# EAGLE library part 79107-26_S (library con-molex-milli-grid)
RECEPTACAL
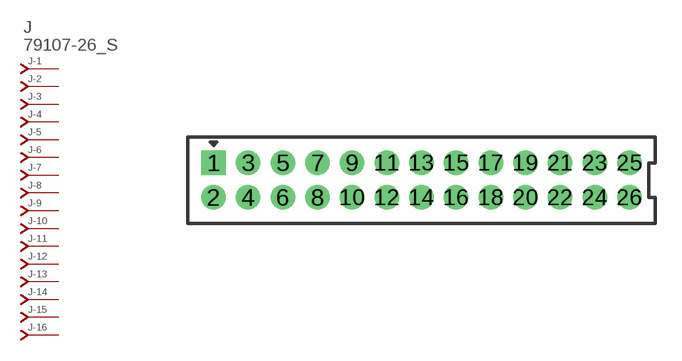
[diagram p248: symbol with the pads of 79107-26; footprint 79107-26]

Designator prefix J; gates -1=J-NV -2=J-N -3=J-N -4=J-N -5=J-N -6=J-N -7=J-N -8=J-N -9=J-N -10=J-N -11=J-N -12=J-N -13=J-N -14=J-N -15=J-N -16=J-N -17=J-N -18=J-N -19=J-N -20=J-N -21=J-N -22=J-N -23=J-N -24=J-N -25=J-N -26=J-N

## 79107-26_S  [79107-26]
1  -1:J  pas
2  -2:J  pas
3  -3:J  pas
4  -4:J  pas
5  -5:J  pas
6  -6:J  pas
7  -7:J  pas
8  -8:J  pas
9  -9:J  pas
10  -10:J  pas
11  -11:J  pas
12  -12:J  pas
13  -13:J  pas
14  -14:J  pas
15  -15:J  pas
16  -16:J  pas
17  -17:J  pas
18  -18:J  pas
19  -19:J  pas
20  -20:J  pas
21  -21:J  pas
22  -22:J  pas
23  -23:J  pas
24  -24:J  pas
25  -25:J  pas
26  -26:J  pas

## Footprint 79107-26 (pad centres in mm)
RECEPTACAL Dual Row, Vertical, Through-Hole
drill 0.914 square: 1 -12,1
drill 0.914: 2 -12,-1; 3 -10,1; 4 -10,-1; 5 -8,1; 6 -8,-1; 7 -6,1; 8 -6,-1; 9 -4,1; 10 -4,-1; 11 -2,1; 12 -2,-1; 13 0,1; 14 0,-1; 15 2,1; 16 2,-1; 17 4,1; 18 4,-1; 19 6,1; 20 6,-1; 21 8,1; 22 8,-1; 23 10,1; 24 10,-1; 25 12,1; 26 12,-1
